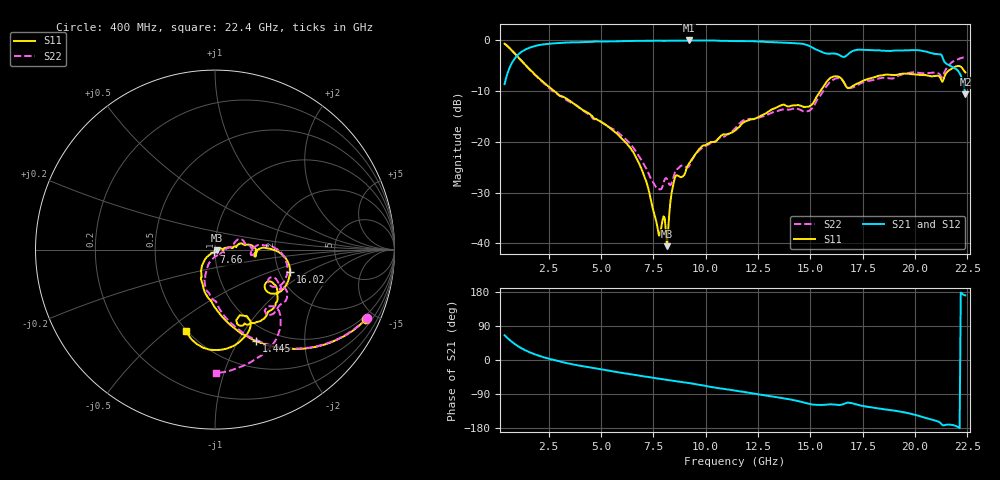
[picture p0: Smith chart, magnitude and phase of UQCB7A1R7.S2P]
!  Part Number  UQCB7A1R7	Mounting Orientation: Vertical
!  Description: RF capacitors
!  Application: Coupling, Bypass, Tuning, DC Block
!  Filters, Matching
# GHZ S DB R 50
! Freq  |S11|  S11 Ph  |S21|  S21 Ph  |S12|  S12 Ph  |S22|  S22 Ph
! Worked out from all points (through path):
!   401 points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, 400 MHz to 22.4 GHz, reference 50 ohm
!   highest |S21| = 0.00 dB at 9.2 GHz (marker M1); lowest = -10.6 dB at 22.4 GHz (marker M2)
!   group delay of S21, straight-line fit = 24.8 ps
!   lowest |S11| = -40.5 dB at 8.155 GHz (marker M3), VSWR 1.02, Z = 50.9 - j0.419 ohm
!   |S11| at or under -10 dB: 2.774 GHz to 15.48 GHz (12.7 GHz wide, 139 % of centre)
!   |S22| runs from -29.3 to -0.6 dB; largest |S21 - S12| = 0.0056
!   S11 on the Smith chart (normalised r, x): 400 MHz: 0.80, -4.45; 1.445 GHz: 0.80, -1.19; 7.66 GHz: 0.99, -0.03; 16.02 GHz: 2.28, -0.70; 22.4 GHz: 0.49, -0.58
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0.4  -0.65 -24.6  -8.61 65.4  -8.62 65.4  -0.65 -24.4
0.84  -2.37 -46.0  -3.82 44.0  -3.83 44.0  -2.36 -45.7
1.445  -5.05 -65.8  -1.67 24.1  -1.69 24.2  -5.09 -65.2
2.435  -8.87 -85.7  -0.69 4.5  -0.70 4.5  -9.05 -83.7
4.085  -13.57 -108.9  -0.34 -15.9  -0.35 -15.9  -13.68 -105.4
6.505  -21.81 -135.2  -0.10 -38.4  -0.09 -38.3  -20.91 -114.0
7.165  -27.82 -135.7  -0.08 -44.1  -0.07 -44.0  -25.22 -105.0
7.66  -36.04 -105.8  -0.04 -48.3  -0.04 -48.2  -29.06 -75.8
7.77  -38.45 -81.5  -0.05 -49.4  -0.05 -49.3  -29.30 -65.4
8.155  -40.53 -26.0  -0.06 -52.5  -0.05 -52.4  -27.30 -46.2
8.54  -26.97 2.5  -0.05 -55.7  -0.04 -55.6  -25.89 -16.2
9.2  -24.30 8.8  0.00 -60.6  -0.01 -60.5  -24.83 -1.0
11.4  -17.74 12.0  -0.12 -80.5  -0.12 -80.5  -17.37 23.8
14.04  -12.92 -5.8  -0.48 -104.2  -0.47 -104.3  -13.60 -4.1
15.085  -12.55 -0.7  -1.36 -117.4  -1.35 -117.5  -13.36 2.9
16.02  -7.23 -16.6  -2.57 -117.0  -2.57 -117.3  -7.93 -9.4
16.845  -9.40 -33.0  -2.55 -112.7  -2.54 -112.9  -9.34 -30.0
18.77  -6.75 -47.1  -2.09 -131.5  -2.08 -131.8  -7.48 -31.8
19.98  -6.67 -61.8  -1.90 -144.4  -1.89 -144.6  -6.27 -36.5
21.19  -7.26 -73.4  -2.71 -165.3  -2.71 -165.5  -6.75 -51.6
21.685  -5.71 -72.4  -5.01 -170.7  -5.03 -171.0  -4.58 -53.5
22.4  -6.30 -109.7  -10.59 170.5  -10.59 170.3  -3.25 -89.8
